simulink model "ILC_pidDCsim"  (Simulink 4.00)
settings: Solver=ode45  SolverMode=SingleTasking  StartTime=time_ILC(1)  StopTime=time_ILC(end)  RelTol=1e-3  AbsTol=1e-6
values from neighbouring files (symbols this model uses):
  tsamp_ILC = 0.010    (= 0.01)    [ILC_setup.m]
libraries: cstblocks x2, simulink3 x1

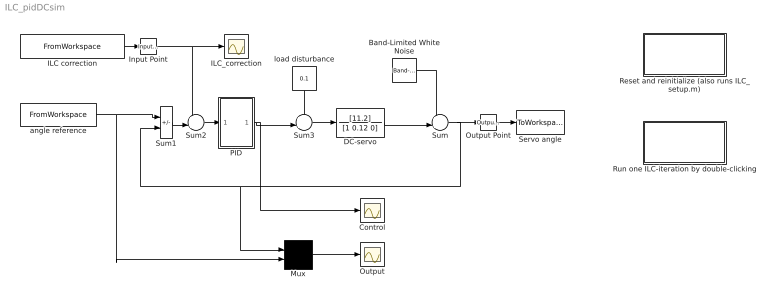
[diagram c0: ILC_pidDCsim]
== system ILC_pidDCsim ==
  Band-Limited White Noise : simulink3/Sources/Band-Limited White Noise  Cov=[0.0001]*0  Ts=0.1  seed=[23341]
  Control : Scope
  DC-servo : TransferFcn  Numerator=[11.2]  Denominator=[1 0.12 0]  AbsoluteTolerance=auto  Realization=auto
  ILC correction : FromWorkspace  VariableName=[ time_ILC correction_ILC(:,idx_ILC)]  SampleTime=tsamp_ILC  OutputAfterFinalValue=Extrapolation
  ILC_correction : Scope
  Input Point : cstblocks/Input Point
  Mux : Mux  Inputs=2
  Output : Scope
  Output Point : cstblocks/Output Point
  PID : Subsystem  mask{K=0.4, Ti=100, Td=0.5}
  Reset and reinitialize (also runs ILC_setup.m) : Subsystem
  Run one ILC-iteration by double-clicking : Subsystem
  Servo angle : ToWorkspace  VariableName=ILC_pos  SampleTime=-1  SaveFormat=StructureWithTime
  Sum : Sum  Inputs=++|  SaturateOnIntegerOverflow=on
  Sum1 : Sum  Inputs=+-  SaturateOnIntegerOverflow=on
  Sum2 : Sum  Inputs=++|  SaturateOnIntegerOverflow=on
  Sum3 : Sum  Inputs=++|  SaturateOnIntegerOverflow=on
  angle reference : FromWorkspace  VariableName=[ time_ILC pos_Reference_ILC]  SampleTime=tsamp_ILC  OutputAfterFinalValue=Extrapolation
  load disturbance : Constant  Orientation=down  Value=0.1
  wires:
  Mux/1 -> Output/1
  PID/1(Out1) -> Control/1, Sum3/2
  DC-servo/1 -> Sum/2
  Sum/1 -> Mux/1, Sum1/2, Output Point/1
  Band-Limited White Noise/1 -> Sum/1
  Output Point/1 -> Servo angle/1
  Sum2/1 -> PID/1(In1)
  Sum1/1 -> Sum2/2
  Sum3/1 -> DC-servo/1
  angle reference/1 -> Mux/2, Sum1/1
  load disturbance/1 -> Sum3/1
  ILC correction/1 -> Input Point/1
  Input Point/1 -> ILC_correction/1, Sum2/1

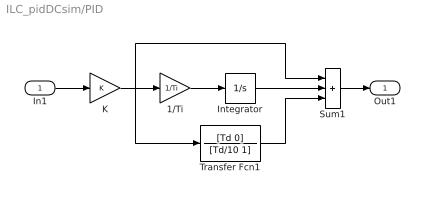
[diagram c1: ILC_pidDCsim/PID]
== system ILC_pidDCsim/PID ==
  In1 : Inport  Port=1  LatchInput=off
  1/Ti : Gain  Gain=1/Ti  Multiplication=Element-wise(K.*u)  SaturateOnIntegerOverflow=on
  Integrator : Integrator  ExternalReset=none  InitialConditionSource=internal  InitialCondition=0  LimitOutput=off  UpperSaturationLimit=inf  LowerSaturationLimit=-inf  ShowSaturationPort=off  ShowStatePort=off  AbsoluteTolerance=auto
  K : Gain  Gain=K  Multiplication=Element-wise(K.*u)  SaturateOnIntegerOverflow=on
  Sum1 : Sum  Inputs=+++  SaturateOnIntegerOverflow=on
  Transfer Fcn1 : TransferFcn  Numerator=[Td 0]  Denominator=[Td/10 1]  AbsoluteTolerance=auto  Realization=auto
  Out1 : Outport  Port=1
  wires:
  In1/1 -> K/1
  K/1 -> 1/Ti/1, Transfer Fcn1/1, Sum1/1
  1/Ti/1 -> Integrator/1
  Sum1/1 -> Out1/1
  Integrator/1 -> Sum1/2
  Transfer Fcn1/1 -> Sum1/3

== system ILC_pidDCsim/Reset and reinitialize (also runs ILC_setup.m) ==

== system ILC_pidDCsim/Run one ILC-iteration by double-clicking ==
